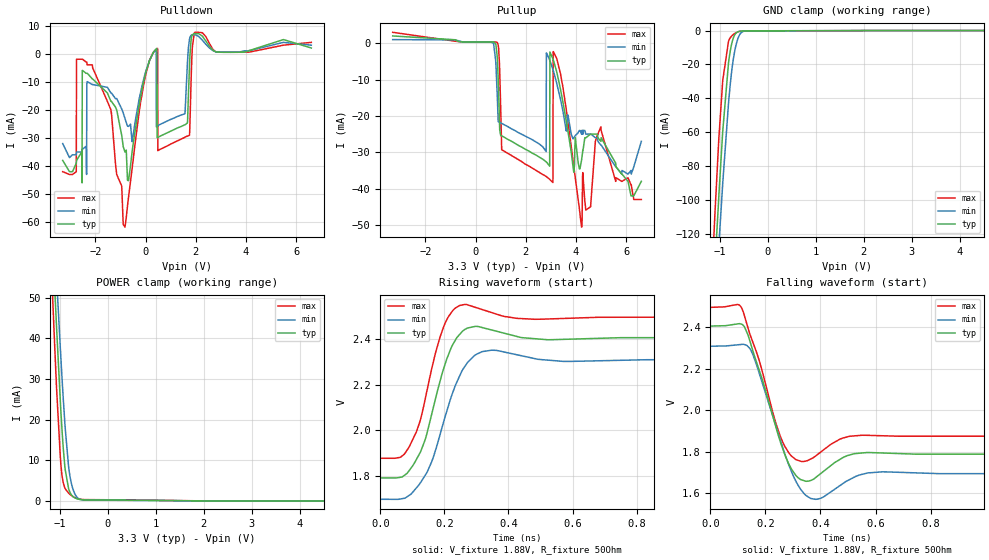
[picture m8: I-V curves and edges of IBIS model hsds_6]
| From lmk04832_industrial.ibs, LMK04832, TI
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|   hsds_6 Model
[Model]   hsds_6
Model_type   3-state
Polarity   Non-Inverting
Vmeas = 2.1
Vref = 1.88
Cref = 1pF
Rref = 50
|   typ   min   max
C_comp   2.136pF   2.117pF   2.176pF
|  Where Nom  PVT is Nominal Process,   3.3V,  25C
|   Fast PVT is Strong Process,   3.45V, -40C
|   Slow PVT is Weak Process,   3.15V, 85C
[Voltage Range]   3.3   3.15   3.45
|Junction Temperature
[Temperature Range]   25   85   -40
[Pullup Reference]   3.3   3.15   3.45
[Pulldown Reference]   0   0   0
[Power Clamp Reference]   3.3   3.15   3.45
[GND Clamp Reference]   0   0   0
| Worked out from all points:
|   GND clamp passes 1 mA (typ) near -0.64 V on its own axis
|   POWER clamp passes 1 mA (typ) near -0.71 V on its own axis
|   falling waveform, V_fixture 1.88V, R_fixture 50Ohm: 20-80 % time 84.2ps typ, 87.7ps min, 82.4ps max; typ from 2.41 V to 1.79 V
|   rising waveform, V_fixture 1.88V, R_fixture 50Ohm: 20-80 % time 72.5ps typ, 84.3ps min, 64.2ps max; typ from 1.79 V to 2.41 V
[Pulldown]
|   Voltage   I(typ)   I(min)   I(max)
-3.3V     -38mA      -32mA      -42mA
-2.76V    -39mA      -36mA      -42mA
-2.75V    -38mA      -35mA      -2mA
-2.53V    -46mA      -34mA      -2mA
-2.52V    -6mA       -34mA      -2mA
-820mV    -35mA      -23.1mA    -61.74mA
320mV     574uA      444uA      607uA
480mV     -29.86mA   -25.77mA   1.855mA
490mV     -29.86mA   -25.67mA   -34.55mA
1.75V     -4.116mA   5.19mA     -29.02mA
1.95V     7.159mA    6.711mA    7.484mA
6.6V      2mA        3mA        4mA
[GND Clamp]
|   Voltage   I(typ)   I(min)   I(max)
-3.3V     -1.535A    -1.479A    -1.61A
-1.52V    -370mA     -382mA     -361mA
-1.1V     -137mA     -164mA     -106mA
-1.09V    -132mA     -159mA     -101mA
-1.03V    -102mA     -131mA     -68.1mA
-1.02V    -96.6mA    -126mA     -63mA
-940mV    -59.2mA    -89.9mA    -29.3mA
-800mV    -15mA      -36.6mA    -5.02mA
-720mV    -4.43mA    -16.9mA    -2.35mA
-620mV    -719uA     -4.45mA    -754uA
-400mV    -186uA     -179uA     -203uA
6.6V      0A         0A         0A
[Pullup]
|   Voltage   I(typ)   I(min)   I(max)
-3.3V     2mA        1mA        3mA
860mV     -3.552mA   -13.76mA   240uA
1.04V     -25.47mA   -22.04mA   -29.31mA
2.81V     -32.62mA   -29.82mA   -36.63mA
2.82V     -32.72mA   -2.646mA   -36.73mA
2.95V     -33.82mA   -4.609mA   -37.43mA
2.96V     -2.407mA   -4.779mA   -37.53mA
3.08V     -4.321mA   -7.213mA   -38.32mA
3.09V     -4.51mA    -7.443mA   -2.299mA
4.22V     -32.2mA    -25mA      -50.6mA
4.99V     -27mA      -28mA      -23mA
6.6V      -38mA      -27mA      -43mA
[POWER Clamp]
|   Voltage   I(typ)   I(min)   I(max)
-3.3V     674mA      627mA      733mA
-1.17V    68.5mA     78.7mA     55.6mA
-1.12V    55.5mA     66.8mA     41.4mA
-1.07V    43mA       55.2mA     28mA
-980mV    22.3mA     35.4mA     9.16mA
-950mV    16.5mA     29.2mA     5.87mA
-890mV    7.82mA     18.1mA     3.07mA
-800mV    2.46mA     6.88mA     1.77mA
-740mV    1.26mA     3.45mA     1.23mA
-670mV    705uA      1.4mA      773uA
-410mV    296uA      245uA      367uA
6.6V      0A         0A         0A
[Ramp]
R_load = 50
|   typ   min   max
dV/dt_r   0.369974/7.1883e-11   0.368119/8.40188e-11   0.372207/6.37286e-11
dV/dt_f   0.369949/8.41217e-11   0.3681/8.73919e-11   0.372177/8.24002e-11
[Falling Waveform]
V_fixture = 1.88V
V_fixture_min = 1.73V
V_fixture_max = 2.03V
R_fixture = 50Ohm
C_fixture = 0F
|   Time   V(typ)   V(min)   V(max)
0s        2.406V     2.309V     2.496V
105.5ps   2.418V     2.317V     2.508V
143.4ps   2.335V     2.298V     2.368V
263.5ps   1.813V     1.818V     1.845V
310.8ps   1.685V     1.658V     1.762V
347.8ps   1.657V     1.589V     1.755V
401.3ps   1.695V     1.576V     1.799V
481.3ps   1.771V     1.646V     1.866V
568.3ps   1.796V     1.696V     1.879V
20ns      1.789V     1.695V     1.876V
[Rising Waveform]
V_fixture = 1.88V
V_fixture_min = 1.73V
V_fixture_max = 2.03V
R_fixture = 50Ohm
C_fixture = 0F
|   Time   V(typ)   V(min)   V(max)
0s        1.789V     1.695V     1.876V
75.22ps   1.801V     1.7V       1.894V
126.3ps   1.907V     1.77V      2.051V
160.7ps   2.072V     1.862V     2.272V
198.1ps   2.272V     2.038V     2.456V
225.4ps   2.375V     2.163V     2.525V
263.5ps   2.443V     2.28V      2.553V
346.7ps   2.441V     2.352V     2.518V
572.6ps   2.4V       2.302V     2.492V
20ns      2.406V     2.309V     2.496V
